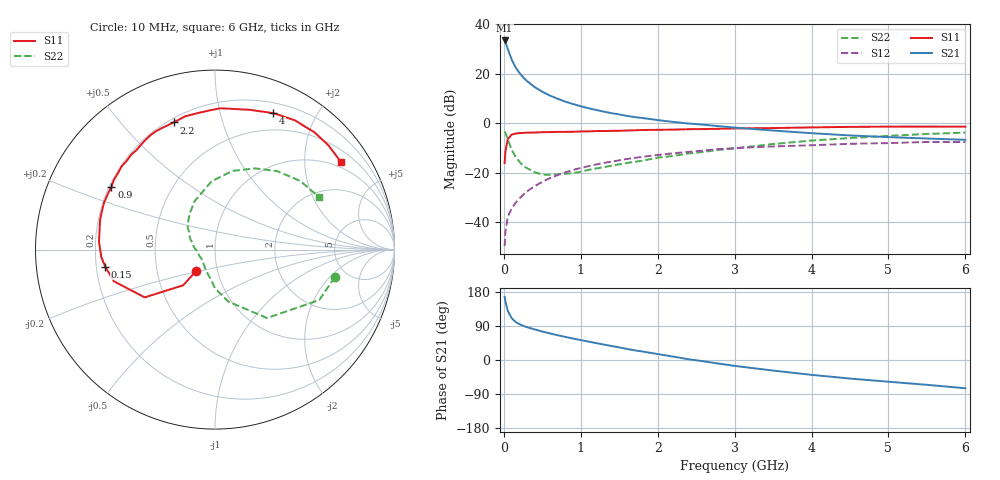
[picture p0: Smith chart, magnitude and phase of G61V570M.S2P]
! SIEMENS Small Signal Semiconductors
! BFG193
! Si NPN RF Bipolar Junction Transistor in SOT223
! VCE = 1.5 V  IC = 70 mA
! Common Emitter S-Parameters:  August  1996
# GHz  S  MA  R  50
!  f  S11  S21  S12  S22
! GHz  MAG  ANG  MAG  ANG  MAG  ANG  MAG  ANG
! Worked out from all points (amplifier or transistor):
!   36 points, 10 MHz to 6 GHz, reference 50 ohm
!   highest |S21| = 33.5 dB at 10 MHz (marker M1)
!   |S21| within 3 dB of that: start of sweep to 46.14 MHz
!   unconditionally stable (mu >= 1): start of sweep to 18.63 MHz; 162.3 MHz to end of sweep
!   at 250 MHz: K = 1.09, MAG = 21.9 dB, |S12| = -28.9 dB
!   at 1.4 GHz: K = 1.13, MAG = 7.6 dB, |S12| = -15.5 dB
!   at 6 GHz: K = 1.03, MAG = -0.6 dB, |S12| = -7.6 dB
!   S11 on the Smith chart (normalised r, x): 10 MHz: 0.79, -0.19; 150 MHz: 0.24, -0.07; 900 MHz: 0.21, +0.27; 2.2 GHz: 0.22, +0.70; 4 GHz: 0.31, +1.47; 6 GHz: 0.82, +2.97
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0.01  0.1576 -131.5  47.17 166.7  0.0033 77.5  0.685 -12.9
0.02  0.2664 -131.7  43.98 155.2  0.0064 67.0  0.6455 -25.8
0.05  0.4734 -145.8  32.07 130.0  0.0126 61.2  0.4788 -52.8
0.1  0.5904 -162.6  19.73 110.9  0.0189 61.9  0.2975 -75.9
0.15  0.6191 -171.2  13.74 100.7  0.0245 63.1  0.2151 -90.1
0.2  0.6349 -176.3  10.57 94.8  0.0301 65.4  0.1692 -97.5
0.25  0.6402 179.6  8.509 90.3  0.0359 66.3  0.1393 -107.3
0.3  0.6479 176.2  7.155 86.6  0.042 67.2  0.1247 -114.0
0.4  0.6521 170.6  5.408 80.8  0.0537 67.7  0.1032 -127.9
0.5  0.6615 165.4  4.338 75.1  0.0658 66.7  0.0923 -139.4
0.6  0.6655 161.2  3.634 70.1  0.0781 65.5  0.091 -148.3
0.7  0.6715 156.9  3.13 65.3  0.0901 64.0  0.0934 -157.4
0.9  0.6746 148.9  2.449 56.6  0.1141 59.8  0.0986 -174.0
1.1  0.6874 142.1  2.017 48.6  0.1363 56.1  0.1149 175.4
1.6  0.7154 125.1  1.412 29.2  0.1902 44.1  0.158 152.9
2.2  0.7451 108.0  1.067 9.0  0.2482 29.3  0.2196 132.4
2.8  0.7754 92.5  0.874 -9.7  0.3013 14.6  0.2912 113.3
3.5  0.8026 76.0  0.715 -27.9  0.3414 -3.6  0.3813 92.8
4  0.8272 66.8  0.632 -39.2  0.3604 -13.5  0.4483 77.7
4.5  0.8466 58.3  0.569 -49.0  0.386 -23.6  0.5042 63.8
5.5  0.8583 42.6  0.493 -65.5  0.4198 -46.5  0.6094 38.9
6  0.8547 35.0  0.465 -74.6  0.4186 -59.5  0.6495 26.9
